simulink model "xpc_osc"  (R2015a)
settings: Solver=ode5  StartTime=0.0  StopTime=2  FixedStep=0.001  RelTol=1e-3
libraries: slrtlib x1

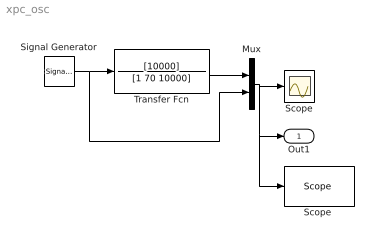
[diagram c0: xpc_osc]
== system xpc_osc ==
  Mux : Mux  Inputs=2
  Scope : Scope
  "Scope " : slrtlib/Displays and Logging/Scope   scopeno=1  scopetype=Target  autostart=on  viewmode=Graphical redraw  formatstr='%15.6f'  grid=on  ylimits=[0,0]  nosamples=2000  noprepostsamples=0  interleave=1  triggermode=FreeRun  triggersignal=1  trigsignalfromport=off  triggerlevel=0.0  triggerslope=Falling  triggerscope=1  triggersample=0  filename=data.dat  mode=Lazy  writesize=512  autorestart=off  dynamicfilemode=off  maxwritefilesize=512*1024^2
  Signal Generator : SignalGenerator  WaveForm=square
  Transfer Fcn : TransferFcn  Numerator=[10000]  Denominator=[1 70 10000]
  Out1 : Outport
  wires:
  Signal Generator/1 -> Transfer Fcn/1, Mux/2
  Transfer Fcn/1 -> Mux/1
  Mux/1 -> "Scope "/1, Out1/1, Scope/1
